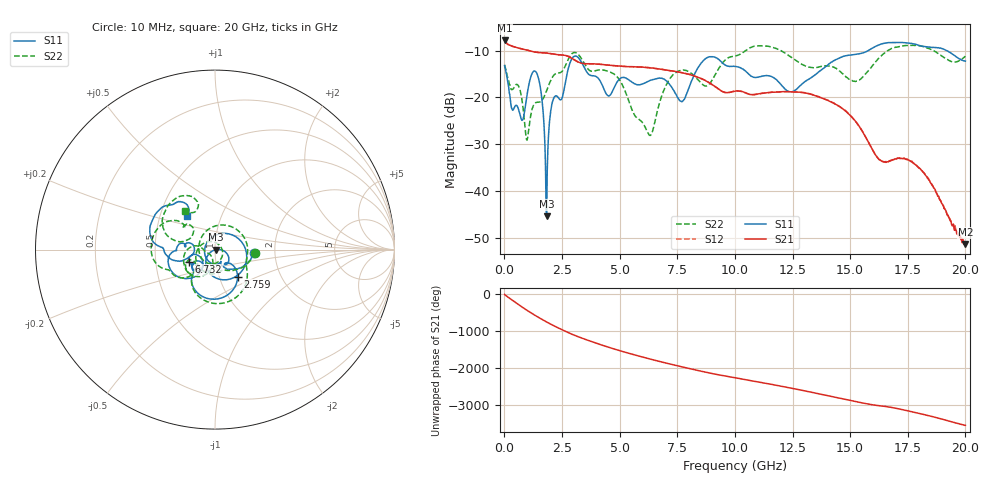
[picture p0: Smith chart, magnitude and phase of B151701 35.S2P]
!  2-Port S-parameters saved by WinCal
! VAR MeasName=S-Parameters (CALIBRATED_DATA) read from VNA (N5244A)
! VAR MeasDate=2015-12-24 19:13:27
! VAR NAME=B151701 35
! VAR FILENAME=B151701 35.S2P
! VAR DATE=2015-12-24 19:13:28
! VAR PHYS_PORTS=1,3
# Hz S DB R 50
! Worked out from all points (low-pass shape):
!   801 points, 10 MHz to 20 GHz, reference 50 ohm
!   highest |S21| = -7.84 dB at 10 MHz (marker M1); lowest = -51.4 dB at 20 GHz (marker M2)
!   |S21| within 3 dB of the highest: start of sweep to 2.258 GHz
!   lowest |S11| = -45.4 dB at 1.834 GHz (marker M3), VSWR 1.01, Z = 50.5 - j0.0324 ohm
!   |S11| at or under -10 dB: start of sweep to 15.79 GHz; 19.18 GHz to end of sweep
!   |S22| runs from -29.1 to -8.9 dB; largest |S21 - S12| = 0.0013
!   S11 on the Smith chart (normalised r, x): 10 MHz: 1.55, -0.06; 2.759 GHz: 1.22, -0.39; 6.732 GHz: 0.74, -0.10; 20 GHz: 0.69, +0.27
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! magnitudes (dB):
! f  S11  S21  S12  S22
! 10 MHz  -13.3  -7.8  -7.8  -13.0
! 759.6 MHz  -24.9  -9.6  -9.6  -20.4
! 984.5 MHz  -19.4  -9.9  -9.9  -29.1
! 1.409 GHz  -14.9  -10.4  -10.4  -21.0
! 1.609 GHz  -19.5  -10.5  -10.5  -20.7
! 1.834 GHz  -45.4  -10.5  -10.5  -18.5
! 2.084 GHz  -21.0  -10.7  -10.7  -15.7
! 2.759 GHz  -14.1  -11.2  -11.2  -12.0
! 3.358 GHz  -12.6  -12.7  -12.7  -11.8
! 4.508 GHz  -19.7  -13.1  -13.1  -14.4
! 6.282 GHz  -16.5  -13.7  -13.6  -28.0
! 6.682 GHz  -15.9  -13.9  -13.9  -22.0
! 6.732 GHz  -15.9  -13.9  -13.9  -21.1
! 7.706 GHz  -20.9  -14.7  -14.7  -14.2
! 8.756 GHz  -11.6  -16.5  -16.5  -17.6
! 10.01 GHz  -13.4  -18.6  -18.6  -11.2
! 12.4 GHz  -18.8  -18.8  -18.7  -11.3
! 13.35 GHz  -15.6  -19.4  -19.4  -13.7
! 15.28 GHz  -10.8  -25.4  -25.3  -16.5
! 16.68 GHz  -8.3  -33.6  -33.7  -9.9
! 18.18 GHz  -9.1  -35.9  -36.0  -9.2
! 20 GHz  -12.3  -51.4  -51.7  -11.2
